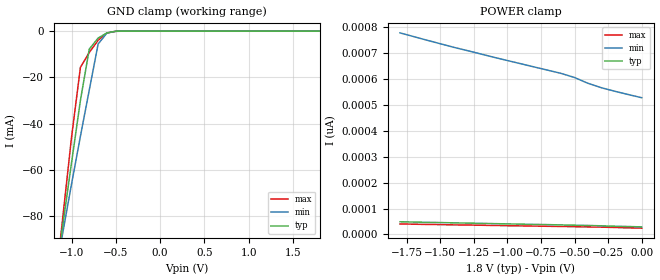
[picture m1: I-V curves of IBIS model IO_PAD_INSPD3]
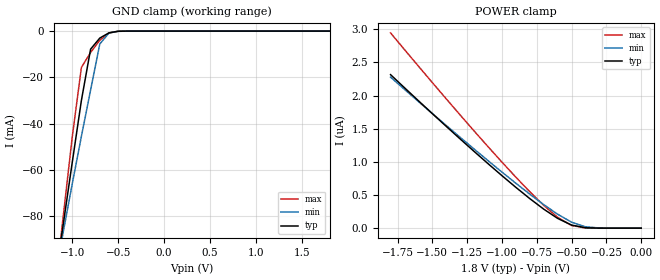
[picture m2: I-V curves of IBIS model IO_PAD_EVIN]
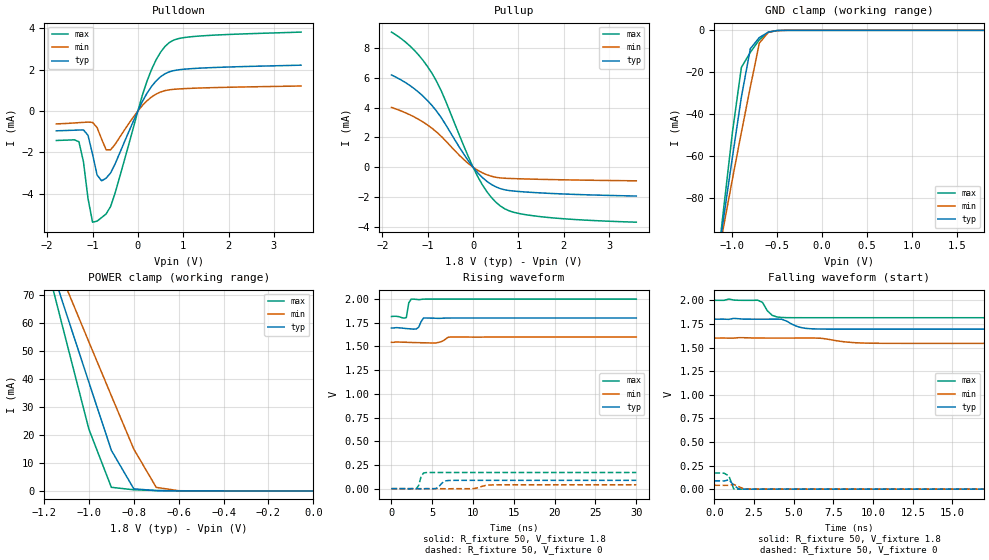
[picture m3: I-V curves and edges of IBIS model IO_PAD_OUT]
[IBIS Ver]   3.2
[Comment Char]   |_char
[File name]   r8804ce_18v.ibs
[File Rev]   1.0
[Date]   2018/09/06 10:15:20
[Source]
[Notes]
[Disclaimer]
This information is for modeling purposes only, and is not guaranteed.
Property of SEIKO EPSON Corp.,
unauthorized reproduction and/or distribution is strictly prohibited.
[Copyright]
Copyright 2018, SEIKO EPSON Corp.
[Component]   r8804ce18v
Si_location Pin
Timing_location Pin
[Manufacturer]   SEIKO EPSON Corp.
| RA/RX-8804CE
[Package]
R_pkg   267m   NA   NA
L_pkg   2.8nH   NA   NA
C_pkg   0.70pF   NA   NA
[Pin] signal_name   model_name
1   FOE   IO_PAD_INSPD3
2   Vdd   POWER
3   EVIN   IO_PAD_EVIN
4   FOUT   IO_PAD_OUT
5   SCL   IO_PAD_INSPD2
6   SOUT   IO_PAD_DIO
7   SDA   IO_PAD_DIO_SMT
8   Vpp   POWER
9   GND   GND
10   /INT   IO_PAD_XINT
| Models and submodels in the file (7): IO_PAD_INSPD3 (Input), IO_PAD_EVIN (Input), IO_PAD_OUT (3-state), IO_PAD_INSPD2 (Input), IO_PAD_DIO (I/O), IO_PAD_DIO_SMT (I/O_open_drain), IO_PAD_XINT (Open_drain)
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[Model]   IO_PAD_INSPD3
Model_type Input
Enable Active-High
Polarity Non-Inverting
Vinh=1.6
Vinl=0.32
C_comp   2.5p   2.0p   3.0p
[Temperature Range] 25   105   -40
[Voltage Range]   1.8   1.6   2.0
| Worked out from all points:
|   GND clamp passes 1 mA (typ) near -0.61 V on its own axis
[GND Clamp]
-1.8V     -278.3mA   -240.3mA   -330mA
-1.2V     -111.6mA   -108.8mA   -116mA
-1.1V     -84.12mA   -87.27mA   -80.81mA
-1V       -56.82mA   -66.05mA   -45.85mA
-900mV    -29.96mA   -45.44mA   -15.68mA
-800mV    -7.804mA   -25.47mA   -9.236mA
-700mV    -3.032mA   -5.585mA   -3.961mA
-600mV    -756.3uA   -818.3uA   -830.7uA
-500mV    -74.57uA   -117.4uA   -45.32uA
1.8V      28.76pA    553.3pA    21.43pA
[POWER Clamp]
-1.8V     48.77pA    779.1pA    40.36pA
-1.4V     44.45pA    723.4pA    36.72pA
-1.1V     41.5pA     684.7pA    34.33pA
-600mV    36.49pA    622.5pA    30.52pA
-500mV    35.41pA    606.5pA    29.62pA
-400mV    34.39pA    584.2pA    28.71pA
-300mV    33.03pA    567pA      27.91pA
-200mV    31.49pA    553.4pA    26.66pA
0V        28.88pA    528.4pA    23.99pA
[Model]   IO_PAD_EVIN
Model_type Input
Enable Active-High
Polarity Non-Inverting
Vinh=1.6
Vinl=0.32
C_comp   2.5p   2.0p   3.0p
[Temperature Range] 25   105   -40
[Voltage Range]   1.8   1.6   2.0
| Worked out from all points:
|   GND clamp passes 1 mA (typ) near -0.61 V on its own axis
[GND Clamp]
-1.8V     -278.3mA   -240.3mA   -330mA
-1.2V     -111.6mA   -108.8mA   -116mA
-1.1V     -84.12mA   -87.27mA   -80.81mA
-1V       -56.82mA   -66.05mA   -45.85mA
-900mV    -29.96mA   -45.44mA   -15.68mA
-800mV    -7.804mA   -25.47mA   -9.236mA
-700mV    -3.032mA   -5.585mA   -3.961mA
-600mV    -756.3uA   -818.3uA   -830.7uA
-500mV    -74.57uA   -117.4uA   -45.32uA
1.8V      28.76pA    723.9pA    21.09pA
[POWER Clamp]
-1.8V     2.316uA    2.279uA    2.946uA
-1.4V     1.536uA    1.549uA    1.951uA
-1V       792.1nA    846.3nA    996.3nA
-800mV    445.9nA    512.7nA    549.4nA
-700mV    286.9nA    355.2nA    343.4nA
-600mV    147.3nA    210nA      163.3nA
-500mV    46.4nA     89.84nA    40.05nA
-400mV    5.964nA    20.38nA    2.634nA
-300mV    372.4pA    2.745nA    85.21pA
0V        28.76pA    528.5pA    23.99pA
[Model]   IO_PAD_OUT
Model_type 3-state
Enable Active-High
Polarity Non-Inverting
Vmeas=0.90
C_comp   2.5p   2.0p   3.0p
[Temperature Range] 25   105   -40
[Voltage Range]   1.8   1.6   2.0
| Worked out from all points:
|   slope of the pulldown table from 0 to 0.27 V, typ, clamps not added: 249 ohm
|   slope of the pullup table from 0 to 0.27 V, typ, clamps not added: 316 ohm
|   GND clamp passes 1 mA (typ) near -0.61 V on its own axis
|   POWER clamp passes 1 mA (typ) near -0.80 V on its own axis
|   falling waveform, R_fixture 50, V_fixture 1.8: 20-80 % time 818ps typ, 1.44ns min, 486ps max; typ from 1.8 V to 1.7 V
|   falling waveform, R_fixture 50, V_fixture 0: 20-80 % time 339ps typ, NA min, 225ps max; typ from 0.088 V to 0 V
|   rising waveform, R_fixture 50, V_fixture 1.8: 20-80 % time 368ps typ, 612ps min, 230ps max; typ from 1.7 V to 1.8 V
|   rising waveform, R_fixture 50, V_fixture 0: 20-80 % time 564ps typ, NA min, 364ps max; typ from 0 V to 0.088 V
[Pullup]
-1.8V     6.186mA    4.013mA    9.06mA
-1.3V     5.273mA    3.375mA    7.854mA
-1.1V     4.756mA    3.025mA    7.148mA
-900mV    4.116mA    2.598mA    6.265mA
-700mV    3.314mA    2.066mA    5.107mA
-200mV    857.2uA    503.2uA    1.393mA
100mV     -362uA     -200uA     -615.4uA
300mV     -933uA     -499.1uA   -1.618mA
600mV     -1.433mA   -714.2uA   -2.593mA
900mV     -1.596mA   -761.3uA   -3.022mA
1.4V      -1.705mA   -803.7uA   -3.28mA
3.6V      -1.929mA   -908.6uA   -3.682mA
[Pulldown]
-1.8V     -961.5uA   -625.3uA   -1.43mA
-1.3V     -922.8uA   -565.9uA   -1.492mA
-1.2V     -918.1uA   -552uA     -2.462mA
-1.1V     -1.178mA   -539uA     -4.238mA
-1V       -2.093mA   -553.4uA   -5.388mA
-900mV    -3.101mA   -801.9uA   -5.336mA
-700mV    -3.256mA   -1.879mA   -4.987mA
-600mV    -2.995mA   -1.879mA   -4.62mA
200mV     855.8uA    491.6uA    1.436mA
600mV     1.806mA    987.6uA    3.13mA
1.2V      2.053mA    1.099mA    3.601mA
3.6V      2.219mA    1.21mA     3.821mA
[GND Clamp]
-1.8V     -299.3mA   -258.9mA   -354mA
-1.2V     -119.5mA   -117.1mA   -123.7mA
-1.1V     -89.88mA   -93.83mA   -85.77mA
-1V       -60.41mA   -70.86mA   -48.66mA
-900mV    -31.76mA   -48.51mA   -17.63mA
-800mV    -8.707mA   -26.99mA   -10.46mA
-700mV    -3.454mA   -6.077mA   -4.512mA
-600mV    -868.8uA   -933.9uA   -956.3uA
-500mV    -86.23uA   -135.8uA   -52.66uA
-400mV    -4.725uA   -14.7uA    -1.074uA
1.8V      21.6pA     5.599nA    11.2pA
[POWER Clamp]
-1.8V     236.4mA    208.9mA    274.8mA
-1.2V     87.98mA    92.05mA    84.88mA
-1.1V     63.38mA    72.67mA    53.4mA
-1V       38.87mA    53.34mA    22.09mA
-900mV    14.53mA    34.09mA    1.297mA
-800mV    753.7uA    14.98mA    407.8uA
-700mV    112.9uA    1.273mA    132.2uA
-600mV    21.58uA    77.12uA    21.07uA
0V        21.6pA     602pA      14.78pA
[Falling Waveform]
R_fixture=50
V_fixture=1.8
V_fixture_min=1.6
V_fixture_max=2.0
0s        1.8V       1.6V       2V
2.727ns   1.8V       1.6V       2.001V
3.03ns    1.8V       1.6V       1.977V
3.333ns   1.8V       1.6V       1.889V
3.636ns   1.8V       1.6V       1.841V
4.242ns   1.799V     1.6V       1.818V
5.455ns   1.712V     1.6V       1.816V
6.364ns   1.697V     1.6V       1.816V
10ns      1.695V     1.545V     1.816V
30ns      1.695V     1.544V     1.816V
[Falling Waveform]
R_fixture=50
V_fixture=0
V_fixture_min=0
V_fixture_max=0
0s        87.71mV    40.74mV    170.6mV
606.1ps   86.1mV     40.09mV    168.5mV
909.1ps   99.16mV    40.37mV    140.8mV
1.212ns   42.22mV    50.39mV    2.776mV
1.515ns   2.823mV    28.16mV    54.52uV
1.818ns   402.5uV    5.153mV    -2.958uV
2.121ns   42.24uV    1.62mV     -18.5uV
2.727ns   -10.67uV   195.2uV    1.286mV
3.03ns    -32.45uV   48.97uV    2.505mV
30ns      0V         0V         0V
[Rising Waveform]
R_fixture=50
V_fixture=1.8
V_fixture_min=1.6
V_fixture_max=2.0
0s        1.695V     1.544V     1.816V
1.818ns   1.689V     1.544V     1.805V
2.121ns   1.687V     1.543V     1.961V
2.424ns   1.685V     1.542V     2V
3.03ns    1.685V     1.541V     1.997V
3.333ns   1.703V     1.54V      1.994V
3.939ns   1.801V     1.539V     1.999V
5.455ns   1.798V     1.537V     2V
7.273ns   1.8V       1.599V     2V
30ns      1.8V       1.6V       2V
[Rising Waveform]
R_fixture=50
V_fixture=0
V_fixture_min=0
V_fixture_max=0
0s        0V         0V         0V
3.03ns    -89.99uV   23.11uV    -2.199mV
3.333ns   -778.6uV   28.21uV    34.37mV
3.636ns   -2.509mV   24.55uV    129.5mV
4.242ns   -11.99uV   23.57uV    169.5mV
5.455ns   1.182mV    -5.61uV    170.5mV
6.97ns    86.15mV    -1.504mV   170.6mV
10ns      87.68mV    301.8uV    170.6mV
12.42ns   87.71mV    39.73mV    170.6mV
30ns      87.71mV    40.74mV    170.6mV
[Ramp]
R_load=50
dV/dt_r   5.262E-2/5.505E-10   2.445E-2/9.509E-10   1.024E-1/3.352E-10
dV/dt_f   6.318E-2/7.892E-10   3.371E-2/1.417E-9   1.106E-1/4.623E-10
|[End   IO_PAD_OUT
